PROGRAM MAIN
VAR
	PMC01 : PMControllerType;	
	PMC01IN AT %IB0 : ARRAY[0..399] OF BYTE;
	PMC01OUT AT %QB0 : ARRAY[0..399] OF BYTE;	
	PMC_AutoRefresh_DB : PMC_AutoRefresh;	
	
	Example01 : Example01_longaxismotion; Example01_run : BOOL; Example01_done : BOOL;	
	Example02 : Example02_shortaxismotion; Example02_run : BOOL; Example02_done : BOOL;
	Example03 : Example03_groups; Example03_run : BOOL; Example03_done : BOOL;
	Example04 : Example04_waituntil; Example04_run : BOOL; Example04_done : BOOL;
	Example05 : Example05_pmccontrol; Example05_run : BOOL; Example05_done : BOOL;
	Example06 : Example06_sync; Example06_run : BOOL; Example06_done : BOOL;
	Example07 : Example07_sun; Example07_run : BOOL; Example07_done : BOOL;
	Example08 : Example08_bufferstatus; Example08_run : BOOL; Example08_done : BOOL;
	Example09 : Example09_groupstatus; Example09_run : BOOL; Example09_done : BOOL;
	Example10 : Example10_waituntiltime; Example10_run : BOOL; Example10_done : BOOL;
	Example11 : Example11_readxbotposition; Example11_run : BOOL;
	Example12 : Example12_DImacro; Example12_run : BOOL; Example12_done : BOOL;
	Example13 : Example13_waituntilDI; Example13_run : BOOL; Example13_done : BOOL;
	Example14 : Example14_DOcmdlb; Example14_run : BOOL; Example14_done : BOOL;
	Example15 : Example15_DOdisplacement; Example15_run : BOOL; Example15_done : BOOL;
	Example16 : Example16_DOmotion; Example16_run : BOOL; Example16_done : BOOL;
	Example17 : Example17_cam; Example17_run : BOOL; Example17_done : BOOL;
	Example18 : Example18_jogging; Example18_run : BOOL; Example18_done : BOOL;
	Example19 : Example19_force; Example19_run : BOOL; Example19_done : BOOL;
	Example20 : Example20_DOforce; Example20_run : BOOL; Example20_done : BOOL;
	Example21 : Example21_startupPMS; Example21_run : BOOL; Example21_done : BOOL;
	Example22 : Example22_stream; Example22_run : BOOL; Example22_done : BOOL;
	Example23 : Example23_holdfor; Example23_run : BOOL; Example23_done : BOOL;
	Example24a : Example24a_autoloading_sending; Example24a_run : BOOL; Example24a_done : BOOL;
	Example24b : Example24b_autoloading_receiving; Example24b_run : BOOL; Example24b_done : BOOL;
	Example25 : Example25_stereotypes; Example25_run : BOOL; Example25_done : BOOL;
	Example26 : Example26_serialnumbers; Example26_run : BOOL; Example26_done : BOOL;
	Example27 : Example27_levitatelandspeed; Example27_run : BOOL; Example27_done : BOOL;
	Example28a : Example28a_zoneunloading; Example28a_run : BOOL; ; Example28a_done : BOOL; Ex28a_UserDone : BOOL; Ex28a_UserStart: BOOL;
	Example28b : Example28b_zoneloading; Example28b_run : BOOL; Example28b_done : BOOL; Ex28b_UserDone : BOOL; Ex28b_UserStart: BOOL;
	Example29 : Example29_recoveryaccident; Example29_run : BOOL; Example29_done : BOOL;
	Example30 : Example30_incoming; Example30_run : BOOL; Example30_done : BOOL;
	Example31 : Example31_extendedfeedback; Example31_run : BOOL;
	Example32 : Example32_zonefencing; Example32_run : BOOL; Example32_done : BOOL;
	Example33 : Example33_StarWheel; Example33_run : BOOL;
	Example34 : Example34_RotaryMotion; Example34_run : BOOL; Example34_done : BOOL;
	Example35 : Example35_Sectors; Example35_run : BOOL; Example35_done : BOOL; Ex35_UserDone : BOOL; Ex35_UserStart : BOOL;
	Example36 : Example36_SetDateAndTime; Example36_run : BOOL; Example36_done : BOOL;
	Example37 : Example37_ApplicationDesigner; Example37_run : BOOL;
END_VAR

//Initialize with location of fieldbus in and out
PMC01.DataFromPMC := ADR(PMC01IN);
PMC01.DataToPMC := ADR(PMC01OUT);
//maintains fieldbus data for PMCLIB to function properly, only needs to by called once per cycle
PMC_AutoRefresh_DB(Enable := TRUE,PM_Controller := PMC01);

//Examples (comment out examples that are not in use to reduce processor load)
Example01(Execute := Example01_run,Done => Example01_done,PM_Controller := PMC01);
//Example02(Execute := Example02_run,Done => Example02_done,PM_Controller := PMC01);
//Example03(Execute := Example03_run,Done => Example03_done,PM_Controller := PMC01);
//Example04(Execute := Example04_run,Done => Example04_done,PM_Controller := PMC01);
//Example05(Execute := Example05_run,Done => Example05_done,PM_Controller := PMC01);
//Example06(Execute := Example06_run,Done => Example06_done,PM_Controller := PMC01);
//Example07(Execute := Example07_run,Done => Example07_done,PM_Controller := PMC01);
//Example08(Execute := Example08_run,Done => Example08_done,PM_Controller := PMC01);
//Example09(Execute := Example09_run,Done => Example09_done,PM_Controller := PMC01);
//Example10(Execute := Example10_run,Done => Example10_done,PM_Controller := PMC01);
//Example11(Execute := Example11_run,PM_Controller := PMC01);
//Example12(Execute := Example12_run,Done => Example12_done,PM_Controller := PMC01);
//Example13(Execute := Example13_run,Done => Example13_done,PM_Controller := PMC01);
//Example14(Execute := Example14_run,Done => Example14_done,PM_Controller := PMC01);
//Example15(Execute := Example15_run,Done => Example15_done,PM_Controller := PMC01);
//Example16(Execute := Example16_run,Done => Example16_done,PM_Controller := PMC01);
//Example17(Execute := Example17_run,Done => Example17_done,PM_Controller := PMC01);
//Example18(Execute := Example18_run,Done => Example18_done,PM_Controller := PMC01);
//Example19(Execute := Example19_run,Done => Example19_done,PM_Controller := PMC01);
//Example20(Execute := Example20_run,Done => Example20_done,PM_Controller := PMC01);
//Example21(Execute := Example21_run,Done => Example21_done,PM_Controller := PMC01);
//Example22(Execute := Example22_run,Done => Example22_done,PM_Controller := PMC01);
//Example23(Execute := Example23_run,Done => Example23_done,PM_Controller := PMC01);
//Example24a(Execute := Example24a_run,Done => Example24a_done,PM_Controller := PMC01);
//Example24b(Execute := Example24b_run,Done => Example24b_done,PM_Controller := PMC01);
//Example25(Execute := Example25_run,Done => Example25_done,PM_Controller := PMC01);
//Example26(Execute := Example26_run,Done => Example26_done,PM_Controller := PMC01);
//Example27(Execute := Example27_run,Done => Example27_done,PM_Controller := PMC01);
//Example28a(Execute := Example28a_run,UserFinishedRemovingXbot := Ex28a_UserDone,UserCanRemoveXbot => Ex28a_UserStart,Done => Example28a_done,PM_Controller := PMC01);
//Example28b(Execute := Example28b_run,UserFinishedAddingXbot := Ex28b_UserDone,UserCanAddXbot => Ex28b_UserStart,Done => Example28b_done,PM_Controller := PMC01);
//Example29(Execute := Example29_run,Done => Example29_done,PM_Controller := PMC01);
//Example30(Execute := Example30_run,Done => Example30_done,PM_Controller := PMC01);
//Example31(Execute := Example31_run,PM_Controller := PMC01);
//Example32(Execute := Example32_run,Done => Example32_done,PM_Controller := PMC01);
//Example33(Execute := Example33_run,PM_Controller := PMC01);
//Example34(Execute := Example34_run,Done => Example34_done,PM_Controller := PMC01);
//Example35(Execute := Example35_run,UserReconnectFinished := Ex35_UserDone,UserCanDisconnectFlyway => Ex35_UserStart,Done => Example35_done,PM_Controller := PMC01);
//Example36(Execute := Example36_run,Done => Example36_done,PM_Controller := PMC01);
//Example37(Execute := Example37_run,PMC := PMC01);

END_PROGRAM
